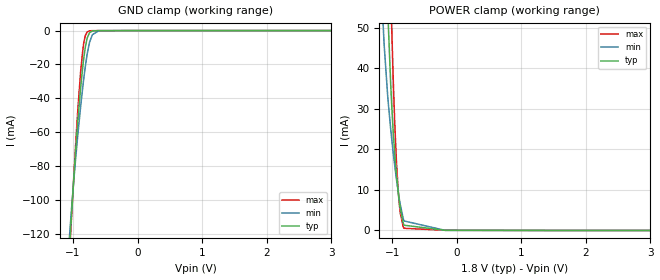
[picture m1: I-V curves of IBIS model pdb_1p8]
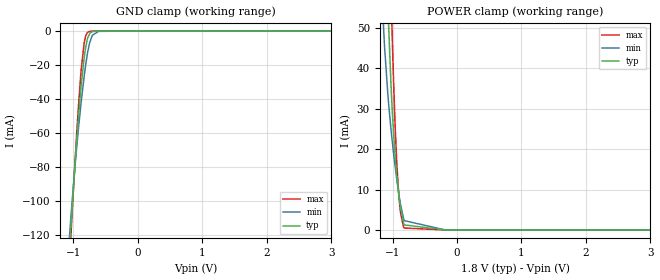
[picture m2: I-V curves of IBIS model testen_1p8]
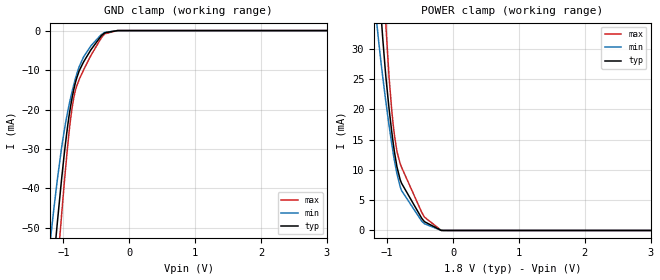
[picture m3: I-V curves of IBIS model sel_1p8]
|Texas Instruments Incorporated
|FPD-Link III 12-bit 100 MHz Deserializer with Selectable Parallel
|or CSI-2 Output
|Marketing part#   Digital Voltage Range   Package-type   #pins
|DS90UB934   1.71 - 3.6   WQFN   48
[IBIS Ver]   4.1
[File name]   ds90ub934_q1.ibs
[File Rev]   1.0
[Date]   5/27/2016
[Source]
| Texas Instruments Incorporated.
| Analog-eLab Design Center, HPA
| 12500 TI Blvd
| Dallas, TX -75243
[Notes]   Revision History:
| Rev 1.0: 5/27/2016
| - Initial version of the model
| - Model generated from simulations in SPECTRE
| - Model matched to SPICE simulation
| - C_comp although listed in numerical order of value are
|   obtained from varying PVT conditions. For PVT conditions for
|   each specific value refer the buffer description under
|   respective [Model]. IBIS model user is responsible for using
|   appropriate C_comp to simulate for Signal Integrity.
[Disclaimer]
| This model is designed as an aid for customers of Texas Instruments.
| TI and its licensors and suppliers make no warranties, either expressed
| or implied, with respect to this  model, including the warranties of
| merchantability or fitness for a particular purpose. The model is
| provided solely on an "as is" basis. The entire risk as to its quality
| and performance is with the customer.
[Copyright]
(C) Copyright 2016 Texas Instruments Incorporated.All rights reserved.
|   DS90UB934_Q1
[Component]   DS90UB934_Q1
[Manufacturer]   TI
[Package]   |48 WQFN
|   typ   min   max
R_pkg  0.042266   0.000540  0.065360
L_pkg  0.707532nH 0.114770nH 1.090470nH
C_pkg  0.120390pF 0.069160pF 0.145430pF
[Pin]  signal_name   model_name   R_pin   L_pin   C_pin
1   I2C_SDA   scl   NA   NA   NA
2   I2C_SCL   scl   NA   NA   NA
3   VDD_1P1_D   power   NA   NA   NA
4   OSS_SEL/XOUT   xout   NA   NA   NA
5   OEN/XIN/REFCLK   xin   NA   NA   NA
6   BISTEN   sel   NA   NA   NA
7   VDDIO   power   NA   NA   NA
8   PCLK/GPIO6   gpio2   NA   NA   NA
9   VSYNC/GPIO5   gpio2   NA   NA   NA
10   HSYNC/GPIO4   gpio2   NA   NA   NA
11   ROUT11/CSI_CLK0N  csi   NA   NA   NA
12   ROUT10/CSI_CLK0P  csi   NA   NA   NA
13   ROUT9/CSI_D0N   csi   NA   NA   NA
14   ROUT8/CSI_D0P   csi   NA   NA   NA
15   ROUT7/CSI_D1N   csi   NA   NA   NA
16   ROUT6/CSI_D1P   csi   NA   NA   NA
17   VDD_1P8   power   NA   NA   NA
18   ROUT5/CSI_CLK1N   csi   NA   NA   NA
19   ROUT4/CSI_CLK1P   csi   NA   NA   NA
20   VDD_1P1_CSI   csi   NA   NA   NA
21   ROUT3/CSI_D2N   csi   NA   NA   NA
22   ROUT2/CSI_D2P   csi   NA   NA   NA
23   ROUT1/CSI_D3N   csi   NA   NA   NA
24   ROUT0/CSI_D3P   csi   NA   NA   NA
25   GPIO3/INTB   gpio2   NA   NA   NA
26   GPIO2   gpio2   NA   NA   NA
27   GPIO1   gpio   NA   NA   NA
28   GPIO0   gpio   NA   NA   NA
29   VDDIO   power   NA   NA   NA
30   PDB   pdb   NA   NA   NA
31   VDD_1P8_FPD1   power   NA   NA   NA
32   RIN1+   rin   NA   NA   NA
33   RIN1-   rin   NA   NA   NA
34   VDD_1P1_FPD   power   NA   NA   NA
35   IDX   pass   NA   NA   NA
36   VDD_1P8_P1   power   NA   NA   NA
37   MODE   mode   NA   NA   NA
38   CMLOUTP   cmlout   NA   NA   NA
39   CMLOUTN   cmlout   NA   NA   NA
40   VDD_1P8_FPD0   power   NA   NA   NA
41   RIN0+   rin   NA   NA   NA
42   RIN0-   rin   NA   NA   NA
43   MIPI_SEL   mipi   NA   NA   NA
44   TESTEN   testen   NA   NA   NA
45   VDD_1P8_P0   power   NA   NA   NA
46   SEL   sel   NA   NA   NA
47   PASS   pass   NA   NA   NA
48   LOCK   pass   NA   NA   NA
49   GND   gnd   NA   NA   NA
[Diff_pin]   inv_pin   vdiff   tdelay_typ   tdelay_min   tdelay_max
32   33   200mV   NA   NA   NA
38   39   NA   NA   NA   NA
41   42   200mV   NA   NA   NA
|   Model Selectors
[Model Selector] pdb
pdb_1p8   1.8V  digital Input
pdb_3p3   3.3V  digital Input
[Model Selector] testen
testen_1p8   1.8V  digital Input
testen_3p3   3.3V  digital Input
[Model Selector] sel
sel_1p8   1.8V  digital Input
sel_3p3   3.3V  digital Input
[Model Selector] xin
xin_1p8   1.8V  digital Input
xin_3p3   3.3V  digital Input
[Model Selector] mipi
mipi_1p8   1.8V  digital Input
mipi_3p3   3.3V  digital Input
[Model Selector] xout
xout_1p8   1.8V  digital Output
xout_3p3   3.3V  digital Output
[Model Selector] pass
pass_1p8   1.8V  digital Output
pass_3p3   3.3V  digital Output
[Model Selector] gpio
gpio_1p8   1.8V  digital Output
gpio_3p3   3.3V  digital Output
[Model Selector] gpio2
gpio2_1p8   1.8V  digital Output
gpio2_3p3   3.3V  digital Output
[Model Selector] scl
scl_1p8   1.8V  digital I/O_open_drain |1MHz
scl_3p3   3.3V  digital I/O_open_drain |1MHz
scl_fast_1p8  1.8V  digital I/O_open_drain |400kHz
scl_fast_3p3  3.3V  digital I/O_open_drain |400kHz
[Model Selector] csi
csi_1p8   1.8V  digital Output
csi_3p3   3.3V  digital Output
| Models and submodels in the file (27): pdb_1p8 (Input), pdb_3p3 (Input), testen_1p8 (Input), testen_3p3 (Input), sel_1p8 (Input), sel_3p3 (Input), xin_1p8 (Input), xin_3p3 (Input), mipi_1p8 (Input), mipi_3p3 (Input), mode (Input), xout_1p8 (Output), xout_3p3 (Output), scl_1p8 (I/O_open_drain), scl_3p3 (I/O_open_drain), scl_fast_1p8 (I/O_open_drain), scl_fast_3p3 (I/O_open_drain), pass_1p8 (Output), pass_3p3 (Output), gpio_1p8 (I/O), gpio_3p3 (I/O), gpio2_1p8 (I/O), gpio2_3p3 (I/O), csi_1p8 (Output), csi_3p3 (Output), rin (I/O), cmlout (Output)
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|   pdb_1p8 Model
[Model]   pdb_1p8
Model_type   Input
Vinl = 0.63
Vinh = 1.17
|   typ   min   max
|   (nom PVT)   (fast PVT)   (slow PVT)
C_comp   3.865e-13   2.951e-13   4.797e-13
| Where nom  PVT is Nominal Process, 1.8V, 27C
|   Fast PVT is Strong Process,  1.89V, -40C
|   Slow PVT is Weak Process,   1.71V, 125C
[Voltage Range]   1.8   1.71   1.89
|Junction Temperature
[Temperature Range]   27   125   -40
[Power Clamp Reference]   1.8   1.71   1.89
[GND Clamp Reference]   0   0   0
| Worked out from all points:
|   GND clamp passes 1 mA (typ) near -0.73 V on its own axis
[GND Clamp]
|   Voltage   I(typ)   I(min)   I(max)
-1.8V     -664.9mA   -592mA     -720.2mA
-1.05V    -125.1mA   -118.5mA   -128.9mA
-1.022V   -107.6mA   -104.5mA   -109.1mA
-936mV    -58.42mA   -65.56mA   -52.56mA
-880mV    -32.68mA   -43.91mA   -23.13mA
-830.4mV  -15.22mA   -27.21mA   -6.421mA
-809.9mV  -9.815mA   -21.18mA   -2.934mA
-779.4mV  -4.24mA    -13.46mA   -743uA
-743.2mV  -1.201mA   -6.745mA   -145.2uA
-700.5mV  -235.6uA   -2.414mA   -38.09uA
-604.7mV  -21.19uA   -171.7uA   -20.72uA
3.6V      0A         0A         0A
[POWER Clamp]
|   Voltage   I(typ)   I(min)   I(max)
-1.8V     575.8mA    438.5mA    682.1mA
-1.178V   116.2mA    62.45mA    168.4mA
-1.127V   85.19mA    46.23mA    130mA
-1.058V   49.79mA    30.88mA    81.36mA
-1.006V   30.25mA    22.24mA    48.75mA
-962.7mV  19.14mA    16.13mA    27.06mA
-933mV    13.48mA    12.4mA     16.28mA
-902.2mV  8.74mA     8.938mA    8.587mA
-876.6mV  5.575mA    6.427mA    4.401mA
-818.5mV  1.296mA    2.351mA    538.9uA
-180mV    39.56uA    32.49uA    49.32uA
3.6V      0A         0A         0A
|   testen_1p8 Model
[Model]   testen_1p8
Model_type   Input
Vinl = 0.63
Vinh = 1.17
|   typ   min   max
|   (nom PVT)   (fast PVT)   (slow PVT)
C_comp   3.223e-13   2.170e-13   4.378e-13
| Where nom  PVT is Nominal Process, 1.8V, 27C
|   Fast PVT is Strong Process,  1.89V, -40C
|   Slow PVT is Weak Process,   1.71V, 125C
[Voltage Range]   1.8   1.71   1.89
|Junction Temperature
[Temperature Range]   27   125   -40
[Power Clamp Reference]   1.8   1.71   1.89
[GND Clamp Reference]   0   0   0
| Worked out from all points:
|   GND clamp passes 1 mA (typ) near -0.73 V on its own axis
[GND Clamp]
|   Voltage   I(typ)   I(min)   I(max)
-1.8V     -652.8mA   -581.4mA   -709.5mA
-1.064V   -132.4mA   -122.9mA   -139.4mA
-1.044V   -119.9mA   -112.7mA   -125.2mA
-1.025V   -108.3mA   -103.4mA   -112.1mA
-936mV    -57.93mA   -63.63mA   -53.19mA
-877.7mV  -31.64mA   -41.63mA   -22.47mA
-828.5mV  -14.73mA   -25.59mA   -6.169mA
-777.5mV  -4.063mA   -12.37mA   -719.8uA
-744.9mV  -1.325mA   -6.544mA   -161.9uA
-703.9mV  -282.5uA   -2.402mA   -31.03uA
-606.4mV  -11.98uA   -164.7uA   -7.929uA
3.6V      0A         0A         0A
[POWER Clamp]
|   Voltage   I(typ)   I(min)   I(max)
-1.8V     575.7mA    438.5mA    682mA
-1.178V   116.1mA    62.4mA     168.3mA
-1.127V   85.13mA    46.18mA    129.9mA
-1.058V   49.73mA    30.84mA    81.29mA
-1.006V   30.19mA    22.19mA    48.68mA
-962.7mV  19.09mA    16.09mA    27mA
-933mV    13.43mA    12.36mA    16.22mA
-902.2mV  8.689mA    8.895mA    8.524mA
-876.6mV  5.525mA    6.385mA    4.339mA
-818.5mV  1.246mA    2.31mA     477.6uA
-180mV    1.965uA    1.563uA    2.529uA
3.6V      0A         0A         0A
|   sel_1p8 Model
[Model]   sel_1p8
Model_type   Input
Vinl = 0.63
Vinh = 1.17
|   typ   min   max
|   (nom PVT)   (fast PVT)   (slow PVT)
C_comp   3.874e-13   3.836e-13   4.472e-13
| Where nom  PVT is Nominal Process, 1.8V, 27C
|   Fast PVT is Strong Process,  1.89V, -40C
|   Slow PVT is Weak Process,   1.71V, 125C
[Voltage Range]   1.8   1.71   1.89
|Junction Temperature
[Temperature Range]   27   125   -40
[Power Clamp Reference]   1.8   1.71   1.89
[GND Clamp Reference]   0   0   0
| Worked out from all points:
|   GND clamp passes 1 mA (typ) near -0.40 V on its own axis
[GND Clamp]
|   Voltage   I(typ)   I(min)   I(max)
-1.8V     -186.8mA   -154.6mA   -219.7mA
-1.184V   -65.39mA   -50.91mA   -80.03mA
-1.142V   -57.47mA   -44.58mA   -70.68mA
-1.093V   -48.73mA   -37.8mA    -60.24mA
-1.032V   -38.29mA   -30.14mA   -47.52mA
-918mV    -21.99mA   -19.11mA   -26.28mA
-867.6mV  -16.94mA   -15.37mA   -19.43mA
-826.6mV  -13.75mA   -12.69mA   -15.72mA
-692.5mV  -7.887mA   -6.617mA   -9.907mA
-371.2mV  -556.6uA   -460.1uA   -816.8uA
-180mV    -2.109uA   -5.617uA   -1.135uA
3.6V      0A         0A         0A
[POWER Clamp]
|   Voltage   I(typ)   I(min)   I(max)
-1.8V     199.4mA    149.9mA    249.5mA
-1.155V   47.02mA    33.97mA    66.22mA
-1.078V   33.32mA    26.3mA     46.84mA
-1.018V   25.07mA    21.03mA    33.44mA
-970.3mV  19.98mA    17.23mA    25.1mA
-930.6mV  16.27mA    14.28mA    19.82mA
-889mV    12.91mA    11.49mA    15.64mA
-851.4mV  10.48mA    9.342mA    13.01mA
-783.2mV  7.824mA    6.611mA    10.47mA
-433.5mV  1.447mA    1.108mA    2.203mA
-180mV    10.65uA    19.17uA    12.51uA
3.6V      0A         0A         0A
